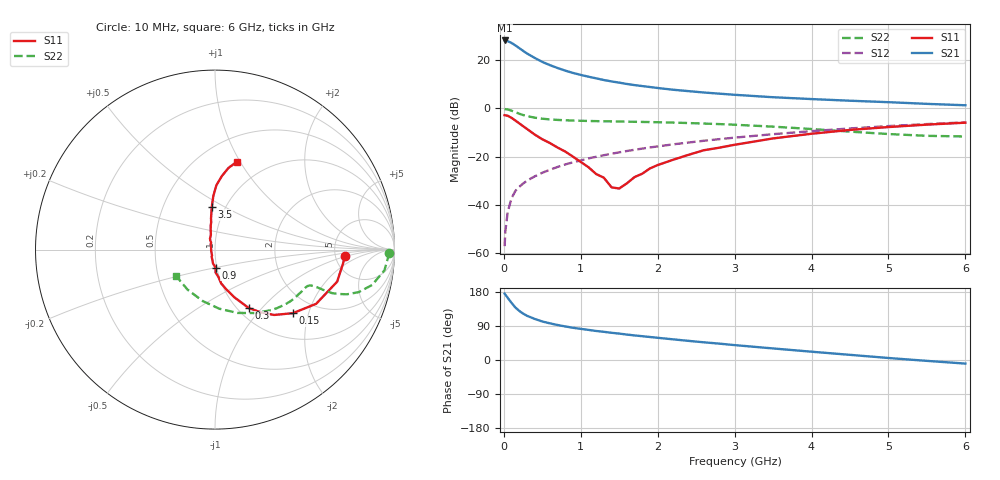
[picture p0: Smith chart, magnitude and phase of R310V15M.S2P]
! SIEMENS Small Signal Semiconductors
! BFR181
! Si NPN RF Bipolar Junction Transistor in SOT23
! VCE = 10 V  IC = 15 mA
! Common Emitter S-Parameters:  May  1996
# GHz  S  MA  R  50
!  f  S11  S21  S12  S22
! GHz  MAG  ANG  MAG  ANG  MAG  ANG  MAG  ANG
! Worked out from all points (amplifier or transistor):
!   36 points, 10 MHz to 6 GHz, reference 50 ohm
!   highest |S21| = 28.2 dB at 10 MHz (marker M1)
!   |S21| within 3 dB of that: start of sweep to 193 MHz
!   unconditionally stable (mu >= 1): 767.9 MHz to 2.744 GHz
!   at 250 MHz: K = 0.68, MSG = 27.5 dB, |S12| = -31.2 dB
!   at 1.4 GHz: K = 1.05, MAG = 13.6 dB, |S12| = -18.8 dB
!   at 6 GHz: K = 0.87, MSG = 3.5 dB, |S12| = -5.8 dB
!   S11 on the Smith chart (normalised r, x): 10 MHz: 6.10, -0.90; 150 MHz: 1.54, -1.59; 300 MHz: 1.12, -0.85; 900 MHz: 0.99, -0.20; 3.5 GHz: 0.86, +0.44; 6 GHz: 0.74, +0.97
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0.01  0.7235 -2.8  25.59 175.1  0.0014 69.3  0.9698 -1.0
0.02  0.7188 -5.7  25.18 172.5  0.0029 77.5  0.9649 -2.7
0.05  0.7037 -14.7  24.77 164.2  0.0071 79.6  0.9511 -7.0
0.1  0.6394 -28.2  22.72 150.7  0.0138 76.5  0.897 -12.7
0.15  0.5602 -39.2  20.16 138.5  0.0195 72.8  0.8348 -16.5
0.2  0.4909 -47.9  17.8 129.7  0.0237 71.4  0.7765 -18.7
0.25  0.4291 -54.2  15.61 122.5  0.0277 69.3  0.7303 -19.8
0.3  0.3767 -59.9  13.8 116.8  0.0318 69.7  0.6948 -20.4
0.4  0.2881 -67.8  11.15 108.5  0.039 69.6  0.6441 -20.4
0.5  0.2295 -74.2  9.201 101.6  0.0465 70.7  0.6116 -20.3
0.6  0.1912 -79.7  7.871 96.7  0.0536 71.3  0.5914 -20.2
0.7  0.1541 -82.8  6.864 92.3  0.0614 71.4  0.5778 -20.4
0.9  0.0999 -88.2  5.43 85.0  0.0766 71.2  0.5607 -21.0
1.1  0.0606 -103.4  4.544 79.5  0.0921 71.1  0.5494 -22.2
1.3  0.0367 -116.9  3.878 74.4  0.1073 70.6  0.5417 -23.9
1.5  0.0219 -167.5  3.42 69.7  0.1231 69.4  0.5353 -26.1
1.7  0.0379 129.3  3.04 64.8  0.1392 68.4  0.528 -28.1
2.2  0.0863 105.5  2.439 54.5  0.18 65.0  0.5082 -34.7
3.5  0.239 94.3  1.705 30.5  0.2926 53.9  0.4192 -57.5
4.5  0.3582 88.8  1.443 13.6  0.3848 43.1  0.3303 -85.8
5.5  0.4616 80.6  1.243 -2.3  0.4739 30.8  0.2704 -124.4
6  0.5063 75.8  1.162 -9.5  0.5152 24.0  0.2624 -146.5
